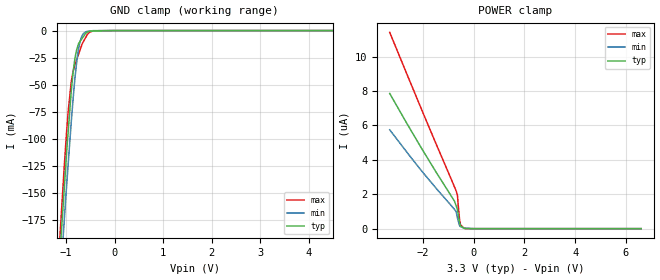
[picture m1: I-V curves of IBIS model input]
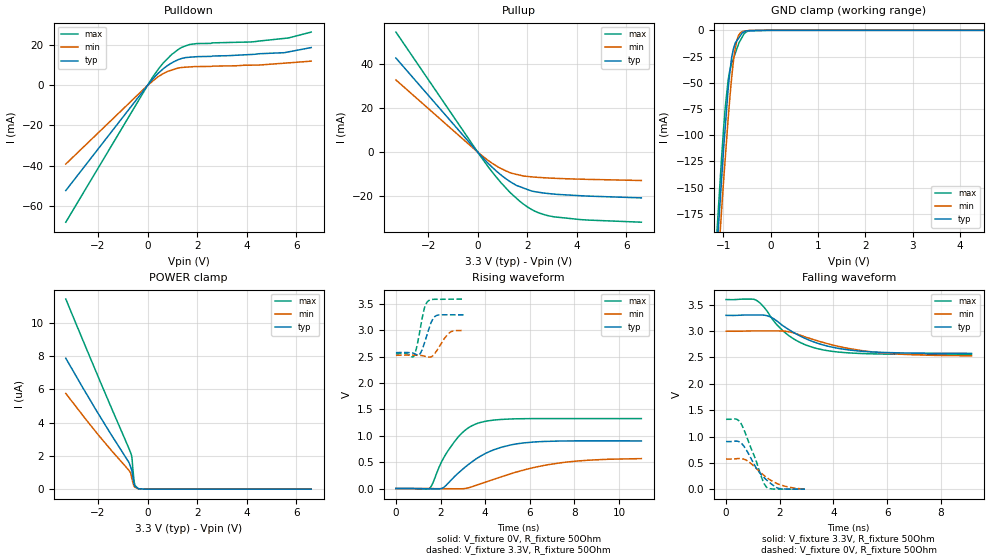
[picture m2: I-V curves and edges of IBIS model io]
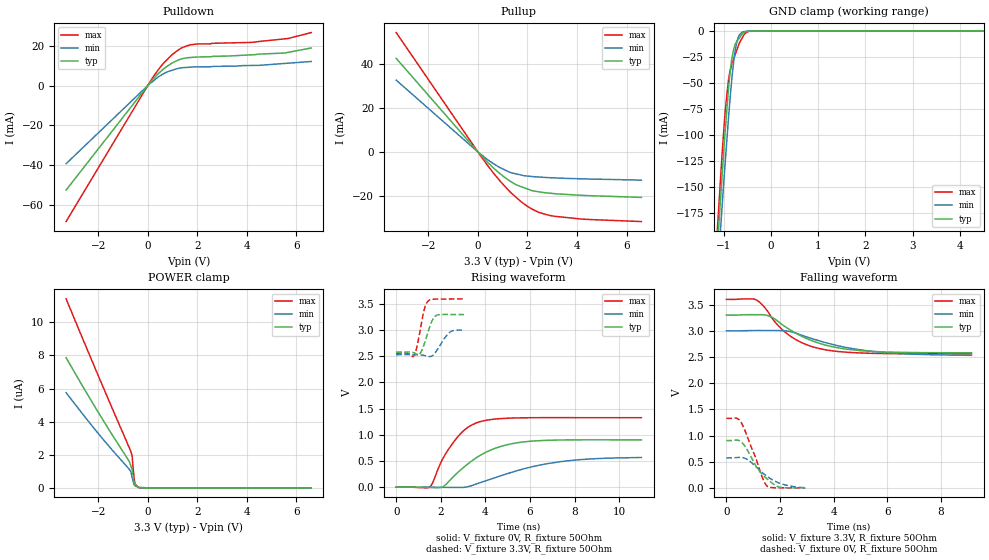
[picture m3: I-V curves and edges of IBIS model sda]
|Texas Instruments Incorporated
| 4ch/4ch Audio CODEC with 2Vrms Driver
| Marketing part#   Digital Voltage Range   Package-type   #pins
| PCM5310PAP   3.0V - 3.6V   HTQFP   64
| PCM5310PAPR   3.0V - 3.6V   HTQFP   64
[IBIS Ver]   3.2
[File name]   pcm5310.ibs
|SIMDE Ver   V3.0 - 201101 - RHL4 - Build 457
[File Rev]   1.0
[Date]   9/16/2011
[Source]
| Texas Instruments Incorporated.
| Analog-eLab Design Center, HPA
| 12500 TI Blvd
| Dallas, TX -75243
| e-mail: elab_scm_ibis@list.ti.com
[Notes]   Revision History:
| Rev 1.0: 9/16/2011
| - Initial version of the model
| - Model generated from simulations in TISPICE
| - Model matched to SPICE simulation
| - C_comp although listed in numerical order of value are
|   obtained from varying PVT conditions. For PVT conditions for
|   each specific value refer the buffer description under
|   respective [Model]. IBIS model user is responsible for using
|   appropriate C_comp to simulate for Signal Integrity.
[Disclaimer]
| This model is designed as an aid for customers of Texas Instruments.
| TI and its licensors and suppliers make no warranties, either expressed
| or implied, with respect to this  model, including the warranties of
| merchantability or fitness for a particular purpose. The model is
| provided solely on an "as is" basis. The entire risk as to its quality
| and performance is with the customer.
[Copyright]
 (C) Copyright 2011 Texas Instruments Incorporated.All rights reserved.
|   PCM5310
[Component]   PCM5310
[Manufacturer]   TI
[Package]   |64 HTQFP   -  PAP package
|   typ   min   max
R_pkg   0.15059   0.08833   0.17303
L_pkg   4.16735nH   3.79786nH   4.68209nH
C_pkg   0.68531pF   0.64149pF   0.80027pF
[Pin]  signal_name   model_name   R_pin   L_pin   C_pin
1   AIN1L   term   0.17241   4.66114nH  0.68445pF
2   AIN1R   term   0.16334   4.44486nH  0.72657pF
3   AIN2L   term   0.15617   4.26409nH  0.70301pF
4   AIN2R   term   0.15114   4.13963nH  0.68633pF
5   AIN3L   term   0.14796   4.05071nH  0.67300pF
6   AIN3R   term   0.14634   3.98580nH  0.66340pF
7   AIN4L   term   0.14631   3.95904nH  0.65785pF
8   AIN4R   term   0.14774   3.96845nH  0.65206pF
9   AIN5L   term   0.15083   4.02619nH  0.65642pF
10   AIN5R   term   0.15490   4.10975nH  0.66911pF
11   AIN6L   term   0.16036   4.24032nH  0.68311pF
12   AIN6R   term   0.16705   4.38885nH  0.68739pF
13   LO1L   term   0.15416   4.20529nH  0.68478pF
14   LO1R   term   0.15888   4.32238nH  0.70717pF
15   LO2L   term   0.16513   4.46842nH  0.72415pF
16   LO2R   term   0.17298   4.68209nH  0.68428pF
17   HGND   gnd   0.06388   3.97515nH  0.79207pF
18   VCCH   power   0.08669   3.91486nH  0.80765pF
19   HPOL   term   0.15364   4.22709nH  0.71008pF
20   VCCP   power   0.07930   3.59861nH  0.75747pF
21   PGND   gnd   0.05537   3.44453nH  0.77490pF
22   HPOR   term   0.14113   3.90151nH  0.66695pF
23   VCCDA   power   0.05352   3.30534nH  0.75554pF
24   AGNDDA   gnd   0.05323   3.27800nH  0.74902pF
25   VCOMDA   term   0.13754   3.79791nH  0.65288pF
26   AGNDS   gnd   0.07445   3.35983nH  0.70413pF
27   SDA   sda   0.13853   3.86286nH  0.65552pF
28   SCL   input   0.14155   3.94706nH  0.66652pF
29   SCK1   io   0.14535   4.05811nH  0.68452pF
30   BCK1   io   0.15232   4.21482nH  0.70298pF
31   LRCK1   io   0.15959   4.37814nH  0.72133pF
32   DATA1   io   0.17116   4.65573nH  0.68694pF
33   SCK2   io   0.17301   4.67994nH  0.68581pF
34   BCK2   io   0.16288   4.44274nH  0.72684pF
35   LRCK2   io   0.15655   4.27586nH  0.70407pF
36   DATA2   io   0.15089   4.13933nH  0.68651pF
37   SCK3   io   0.14816   4.05722nH  0.67339pF
38   BCK3   io   0.14632   3.98772nH  0.66321pF
39   LRCK3   io   0.14628   3.95934nH  0.65736pF
40   DATA3   io   0.14793   3.97169nH  0.64809pF
41   VDD   power   0.05593   3.39080nH  0.72906pF
42   DGND   gnd   0.05586   3.39760nH  0.74125pF
43   SCK4   io   0.14636   3.99488nH  0.66418pF
44   BCK4   io   0.14816   4.05714nH  0.67293pF
45   LRCK4   io   0.15096   4.15065nH  0.68929pF
46   DATA4   io   0.15661   4.28320nH  0.70608pF
47   SCK5   io   0.16282   4.42770nH  0.72281pF
48   BCK5   io   0.17303   4.68090nH  0.68810pF
49   LRCK5   io   0.17111   4.63717nH  0.68447pF
50   DATA5   io   0.15963   4.37847nH  0.72425pF
51   SCK6   io   0.15226   4.19368nH  0.69988pF
52   BCK6   io   0.14528   4.03450nH  0.68056pF
53   LRCK6   io   0.14153   3.93522nH  0.66613pF
54   DATA6   io   0.13849   3.84502nH  0.65470pF
55   GPIO1   io   0.13758   3.80184nH  0.64811pF
56   GPIO2   io   0.13828   3.79786nH  0.64149pF
57   GPIO3   io   0.14026   3.83554nH  0.64456pF
58   _RSTB   input   0.14434   3.91967nH  0.65643pF
59   AMUTE   input   0.14861   4.02993nH  0.66598pF
60   VCCAD   power   0.05705   3.53301nH  0.77678pF
61   AGNDAD   gnd   0.05818   3.62276nH  0.80355pF
62   VREFAD1   term   0.15708   4.28922nH  0.71633pF
63   VREFAD2   term   0.08833   3.95368nH  0.80027pF
64   VCOMAD   term   0.09223   4.14926nH  0.75899pF
[Model] term
Model_type Terminator
C_comp   1.0e-20F  1.0e-20F  1.0e-20F
|   typ   min   max
[Voltage Range]   3.3V   3.0V   3.6V
[POWER Clamp Reference]   3.3V   3.0V   3.6V
[GND Clamp Reference]   0V   0V   0V
|Ambient Temperature   25   85   -25
|Junction Temperature
[Temperature Range]   33   93   -25
| Models and submodels in the file (4): input (Input), io (I/O), sda (I/O), term (Terminator)
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|   input Model
[Model]   input
Model_type   Input
Vinl = 0.99
Vinh = 2.31
|   typ   min   max
|   (nom PVT)   (fast PVT)   (slow PVT)
C_comp   1.334e-12   1.158e-12   1.561e-12
| Where nom  PVT is Nominal Process, 3.3V, 33C
|   Fast PVT is Strong Process,  3.6V, -25C
|   Slow PVT is Weak Process,   3V, 93C
[Model Spec]
|Subparameter   typ   min   max
Vinh   2.31   2.1   2.52
Vinl   0.99   0.9   1.08
[Voltage Range]   3.3   3   3.6
|Ambient Temperature   25   85   -25
|Junction Temperature
[Temperature Range]   33   93   -25
[Power Clamp Reference]   3.3   3   3.6
[GND Clamp Reference]   0   0   0
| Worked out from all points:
|   GND clamp passes 1 mA (typ) near -0.54 V on its own axis
[GND Clamp]
|   Voltage   I(typ)   I(min)   I(max)
-3.3V     -1.899A    -1.874A    -1.956A
-1.149V   -221.5mA   -249.2mA   -204.1mA
-1.115V   -197mA     -226.3mA   -179.6mA
-1.048V   -150.6mA   -179.9mA   -130.2mA
-961.2mV  -94.27mA   -124.2mA   -75.24mA
-896.4mV  -56.08mA   -84.28mA   -47.17mA
-825mV    -26.82mA   -46.29mA   -31.99mA
-747mV    -12.19mA   -16.97mA   -21.98mA
-681mV    -7.826mA   -5.372mA   -13.54mA
-591mV    -2.011mA   -1.028mA   -5.715mA
-133.2mV  -132.3uA   -1.179uA   -14nA
6.6V      0A         0A         0A
[POWER Clamp]
|   Voltage   I(typ)   I(min)   I(max)
-3.3V     7.861uA    5.747uA    11.41uA
-2.046V   4.67uA     3.363uA    6.933uA
-745.8mV  1.586uA    1.113uA    2.411uA
-702mV    1.4uA      1.02uA     2.256uA
-678mV    1.298uA    947.2nA    2.16uA
-633.6mV  1.11uA     627.7nA    1.923uA
-601.2mV  803nA      442.6nA    1.326uA
-558mV    399.5nA    213.3nA    657nA
-518.4mV  190.8nA    121.1nA    267.6nA
-399.6mV  56.97nA    45.99nA    48.59nA
-133.2mV  0A         12.42nA    0A
6.6V      0A         0A         0A
|   io Model
[Model]   io
Model_type   I/O
Polarity   Non-Inverting
Enable   Active-Low
Vinl = 0.99
Vinh = 2.31
Vmeas = 1.65
Vref = 1.65
Cref = 20pF
Rref = 50
|   typ   min   max
|   (nom PVT)   (fast PVT)   (slow PVT)
C_comp   1.341e-12   1.164e-12   1.575e-12
|C_comp ON   1.391e-12   1.198e-12   1.650e-12
|C_comp High Z   1.292e-12   1.129e-12   1.501e-12
| Where nom  PVT is Nominal Process, 3.3V, 33C
|   Fast PVT is Strong Process,  3.6V, -25C
|   Slow PVT is Weak Process,   3V, 93C
[Model Spec]
|Subparameter   typ   min   max
Vinh   2.31   2.1   2.52
Vinl   0.99   0.9   1.08
[Voltage Range]   3.3   3   3.6
|Ambient Temperature   25   85   -25
|Junction Temperature
[Temperature Range]   33   93   -25
[Pullup Reference]   3.3   3   3.6
[Pulldown Reference]   0   0   0
[Power Clamp Reference]   3.3   3   3.6
[GND Clamp Reference]   0   0   0
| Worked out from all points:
|   slope of the pulldown table from 0 to 0.495 V, typ, clamps not added: 73.3 ohm
|   slope of the pullup table from 0 to 0.495 V, typ, clamps not added: 84.4 ohm
|   GND clamp passes 1 mA (typ) near -0.54 V on its own axis
|   falling waveform, V_fixture 3.3V, R_fixture 50Ohm: 20-80 % time 1.74ns typ, 2.29ns min, 1.33ns max; typ from 3.3 V to 2.58 V
|   rising waveform, V_fixture 0V, R_fixture 50Ohm: 20-80 % time 1.79ns typ, 2.89ns min, 1.18ns max; typ from 0 V to 0.904 V
|   rising waveform, V_fixture 3.3V, R_fixture 50Ohm: 20-80 % time 332ps typ, 442ps min, 284ps max; typ from 2.58 V to 3.29 V
|   falling waveform, V_fixture 0V, R_fixture 50Ohm: 20-80 % time 715ps typ, 863ps min, 575ps max; typ from 0.905 V to 0.001 V
[Pulldown]
|   Voltage   I(typ)   I(min)   I(max)
-3.3V     -52.46mA   -39.23mA   -68.24mA
172.8mV   2.65mA     1.778mA    3.487mA
586.8mV   7.767mA    5.542mA    10.48mA
979.2mV   11.22mA    7.635mA    15.45mA
1.382V    13.42mA    8.913mA    19mA
1.706V    14.03mA    9.196mA    20.41mA
2.578V    14.44mA    9.49mA     21.15mA
4.316V    15.47mA    10.08mA    21.78mA
5.674V    16.66mA    11.2mA     23.61mA
6.6V      18.83mA    12.06mA    26.55mA
[GND Clamp]
|   Voltage   I(typ)   I(min)   I(max)
-3.3V     -1.899A    -1.874A    -1.956A
-1.149V   -221.5mA   -249.2mA   -204.1mA
-1.115V   -197mA     -226.3mA   -179.6mA
-1.048V   -150.6mA   -179.9mA   -130.2mA
-961.2mV  -94.27mA   -124.2mA   -75.24mA
-896.4mV  -56.08mA   -84.28mA   -47.17mA
-825mV    -26.82mA   -46.29mA   -31.99mA
-747mV    -12.19mA   -16.97mA   -21.98mA
-681mV    -7.826mA   -5.372mA   -13.54mA
-591mV    -2.011mA   -1.028mA   -5.715mA
-133.2mV  -132.3uA   -1.179uA   -14nA
6.6V      0A         0A         0A
[Pullup]
|   Voltage   I(typ)   I(min)   I(max)
-3.3V     42.63mA    32.71mA    54.38mA
2.629fV   -176.6pA   -125.3pA   -192.6pA
396mV     -4.786mA   -3.572mA   -6.235mA
882mV     -9.807mA   -7.105mA   -13.09mA
1.246V    -12.9mA    -9.046mA   -17.57mA
1.574V    -15.12mA   -10.09mA   -21mA
1.825V    -16.16mA   -10.75mA   -23.37mA
2.168V    -17.59mA   -11.18mA   -25.92mA
2.473V    -18.19mA   -11.44mA   -27.55mA
3.089V    -19.01mA   -11.83mA   -29.31mA
4.316V    -19.84mA   -12.29mA   -30.67mA
6.6V      -20.71mA   -12.84mA   -31.72mA
[POWER Clamp]
|   Voltage   I(typ)   I(min)   I(max)
-3.3V     7.861uA    5.747uA    11.41uA
-2.046V   4.67uA     3.363uA    6.933uA
-745.8mV  1.586uA    1.113uA    2.411uA
-702mV    1.4uA      1.02uA     2.256uA
-678mV    1.298uA    947.2nA    2.16uA
-633.6mV  1.11uA     627.7nA    1.923uA
-601.2mV  803nA      442.6nA    1.326uA
-558mV    399.5nA    213.3nA    657nA
-518.4mV  190.8nA    121.1nA    267.6nA
-399.6mV  56.97nA    45.99nA    48.59nA
-133.2mV  0A         12.42nA    0A
6.6V      0A         0A         0A
[Ramp]
R_load = 50
|   typ   min   max
dV/dt_r   0.542102/1.79695e-09   0.340537/2.89024e-09   0.796156/1.17807e-09
dV/dt_f   0.432533/1.73934e-09   0.282327/2.30553e-09   0.625868/1.32736e-09
[Falling Waveform]
V_fixture = 3.3V
V_fixture_min = 3V
V_fixture_max = 3.6V
R_fixture = 50Ohm
|   Time   V(typ)   V(min)   V(max)
0s        3.3V       3V         3.6V
1.117ns   3.307V     3.006V     3.589V
1.427ns   3.303V     3.005V     3.446V
1.654ns   3.268V     3.005V     3.281V
2.344ns   3.028V     2.988V     2.913V
2.932ns   2.865V     2.893V     2.745V
3.533ns   2.75V      2.798V     2.653V
4.436ns   2.653V     2.684V     2.592V
5.837ns   2.596V     2.587V     2.565V
9.137ns   2.579V     2.531V     2.558V
[Rising Waveform]
V_fixture = 0V
V_fixture_min = 0V
V_fixture_max = 0V
R_fixture = 50Ohm
|   Time   V(typ)   V(min)   V(max)
0s        58.18uV    37.78uV    65.21uV
1.503ns   -5.332mV   49.14uV    3.119mV
2.112ns   14.01mV    -2.985mV   560.3mV
2.648ns   236mV      -4.539mV   902.6mV
3.169ns   428.9mV    5.399mV    1.129V
3.75ns    604.1mV    84mV       1.25V
4.724ns   782.5mV    222.4mV    1.311V
5.755ns   867.1mV    354.4mV    1.325V
7.72ns    903.1mV    505.4mV    1.328V
11ns      903.6mV    567.6mV    1.327V
[Rising Waveform]
V_fixture = 3.3V
V_fixture_min = 3V
V_fixture_max = 3.6V
R_fixture = 50Ohm
|   Time   V(typ)   V(min)   V(max)
0s        2.579V     2.529V     2.556V
800ps     2.566V     2.53V      2.51V
927ps     2.538V     2.529V     2.677V
1.104ns   2.571V     2.526V     3.064V
1.279ns   2.761V     2.513V     3.426V
1.438ns   2.978V     2.494V     3.556V
1.658ns   3.217V     2.522V     3.589V
1.833ns   3.285V     2.618V     3.591V
2.396ns   3.297V     2.956V     3.593V
3.041ns   3.295V     2.999V     3.595V
[Falling Waveform]
V_fixture = 0V
V_fixture_min = 0V
V_fixture_max = 0V
R_fixture = 50Ohm
|   Time   V(typ)   V(min)   V(max)
0s        904.6mV    572.8mV    1.327V
375ps     913.2mV    578.3mV    1.33V
552ps     879.9mV    581.6mV    1.25V
814ps     694.2mV    532.1mV    933mV
1.097ns   424.4mV    407.9mV    571.9mV
1.193ns   349.6mV    361.2mV    421.4mV
1.383ns   235.7mV    274.5mV    145.7mV
1.51ns    174.6mV    223.3mV    37.75mV
1.951ns   16.82mV    96.63mV    1.803mV
2.938ns   871.3uV    4.641mV    831.5uV
|   sda Model
[Model]   sda
Model_type   I/O
Polarity   Non-Inverting
Enable   Active-Low
Vinl = 0.99
Vinh = 2.31
Vmeas = 1.65
Vref = 1.65
Cref = 400pF
Rref = 50
|   typ   min   max
|   (nom PVT)   (fast PVT)   (slow PVT)
C_comp   1.341e-12   1.164e-12   1.575e-12
|C_comp ON   1.391e-12   1.198e-12   1.650e-12
|C_comp OFF   1.292e-12   1.129e-12   1.501e-12
| Where nom  PVT is Nominal Process, 3.3V, 33C
|   Fast PVT is Strong Process,  3.6V, -25C
|   Slow PVT is Weak Process,   3V, 93C
[Model Spec]
|Subparameter   typ   min   max
Vinh   2.31   2.1   2.52
Vinl   0.99   0.9   1.08
[Voltage Range]   3.3   3   3.6
|Ambient Temperature   25   85   -25
|Junction Temperature
[Temperature Range]   33   93   -25
[Pullup Reference]   3.3   3   3.6
[Pulldown Reference]   0   0   0
[Power Clamp Reference]   3.3   3   3.6
[GND Clamp Reference]   0   0   0
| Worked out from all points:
|   slope of the pulldown table from 0 to 0.495 V, typ, clamps not added: 73.3 ohm
|   slope of the pullup table from 0 to 0.495 V, typ, clamps not added: 84.4 ohm
|   GND clamp passes 1 mA (typ) near -0.54 V on its own axis
|   falling waveform, V_fixture 3.3V, R_fixture 50Ohm: 20-80 % time 1.74ns typ, 2.29ns min, 1.33ns max; typ from 3.3 V to 2.58 V
|   rising waveform, V_fixture 0V, R_fixture 50Ohm: 20-80 % time 1.79ns typ, 2.89ns min, 1.18ns max; typ from 0 V to 0.904 V
|   rising waveform, V_fixture 3.3V, R_fixture 50Ohm: 20-80 % time 332ps typ, 442ps min, 284ps max; typ from 2.58 V to 3.29 V
|   falling waveform, V_fixture 0V, R_fixture 50Ohm: 20-80 % time 715ps typ, 863ps min, 575ps max; typ from 0.905 V to 0.001 V
[Pulldown]
|   Voltage   I(typ)   I(min)   I(max)
-3.3V     -52.46mA   -39.23mA   -68.24mA
172.8mV   2.65mA     1.778mA    3.487mA
586.8mV   7.767mA    5.542mA    10.48mA
979.2mV   11.22mA    7.635mA    15.45mA
1.382V    13.42mA    8.913mA    19mA
1.706V    14.03mA    9.196mA    20.41mA
2.578V    14.44mA    9.49mA     21.15mA
4.316V    15.47mA    10.08mA    21.78mA
5.674V    16.66mA    11.2mA     23.61mA
6.6V      18.83mA    12.06mA    26.55mA
[GND Clamp]
|   Voltage   I(typ)   I(min)   I(max)
-3.3V     -1.899A    -1.874A    -1.956A
-1.149V   -221.5mA   -249.2mA   -204.1mA
-1.115V   -197mA     -226.3mA   -179.6mA
-1.048V   -150.6mA   -179.9mA   -130.2mA
-961.2mV  -94.27mA   -124.2mA   -75.24mA
-896.4mV  -56.08mA   -84.28mA   -47.17mA
-825mV    -26.82mA   -46.29mA   -31.99mA
-747mV    -12.19mA   -16.97mA   -21.98mA
-681mV    -7.826mA   -5.372mA   -13.54mA
-591mV    -2.011mA   -1.028mA   -5.715mA
-133.2mV  -132.3uA   -1.179uA   -14nA
6.6V      0A         0A         0A
[Pullup]
|   Voltage   I(typ)   I(min)   I(max)
-3.3V     42.63mA    32.71mA    54.38mA
2.629fV   -176.6pA   -125.3pA   -192.6pA
396mV     -4.786mA   -3.572mA   -6.235mA
882mV     -9.807mA   -7.105mA   -13.09mA
1.246V    -12.9mA    -9.046mA   -17.57mA
1.574V    -15.12mA   -10.09mA   -21mA
1.825V    -16.16mA   -10.75mA   -23.37mA
2.168V    -17.59mA   -11.18mA   -25.92mA
2.473V    -18.19mA   -11.44mA   -27.55mA
3.089V    -19.01mA   -11.83mA   -29.31mA
4.316V    -19.84mA   -12.29mA   -30.67mA
6.6V      -20.71mA   -12.84mA   -31.72mA
[POWER Clamp]
|   Voltage   I(typ)   I(min)   I(max)
-3.3V     7.861uA    5.747uA    11.41uA
-2.046V   4.67uA     3.363uA    6.933uA
-745.8mV  1.586uA    1.113uA    2.411uA
-702mV    1.4uA      1.02uA     2.256uA
-678mV    1.298uA    947.2nA    2.16uA
-633.6mV  1.11uA     627.7nA    1.923uA
-601.2mV  803nA      442.6nA    1.326uA
-558mV    399.5nA    213.3nA    657nA
-518.4mV  190.8nA    121.1nA    267.6nA
-399.6mV  56.97nA    45.99nA    48.59nA
-133.2mV  0A         12.42nA    0A
6.6V      0A         0A         0A
[Ramp]
R_load = 50
|   typ   min   max
dV/dt_r   0.542102/1.79695e-09   0.340537/2.89024e-09   0.796156/1.17807e-09
dV/dt_f   0.432533/1.73934e-09   0.282327/2.30553e-09   0.625868/1.32736e-09
[Falling Waveform]
V_fixture = 3.3V
V_fixture_min = 3V
V_fixture_max = 3.6V
R_fixture = 50Ohm
|   Time   V(typ)   V(min)   V(max)
0s        3.3V       3V         3.6V
1.117ns   3.307V     3.006V     3.589V
1.427ns   3.303V     3.005V     3.446V
1.654ns   3.268V     3.005V     3.281V
2.344ns   3.028V     2.988V     2.913V
2.932ns   2.865V     2.893V     2.745V
3.533ns   2.75V      2.798V     2.653V
4.436ns   2.653V     2.684V     2.592V
5.837ns   2.596V     2.587V     2.565V
9.137ns   2.579V     2.531V     2.558V
[Rising Waveform]
V_fixture = 0V
V_fixture_min = 0V
V_fixture_max = 0V
R_fixture = 50Ohm
|   Time   V(typ)   V(min)   V(max)
0s        58.18uV    37.78uV    65.21uV
1.503ns   -5.332mV   49.14uV    3.119mV
2.112ns   14.01mV    -2.985mV   560.3mV
2.648ns   236mV      -4.539mV   902.6mV
3.169ns   428.9mV    5.399mV    1.129V
3.75ns    604.1mV    84mV       1.25V
4.724ns   782.5mV    222.4mV    1.311V
5.755ns   867.1mV    354.4mV    1.325V
7.72ns    903.1mV    505.4mV    1.328V
11ns      903.6mV    567.6mV    1.327V
[Rising Waveform]
V_fixture = 3.3V
V_fixture_min = 3V
V_fixture_max = 3.6V
R_fixture = 50Ohm
|   Time   V(typ)   V(min)   V(max)
0s        2.579V     2.529V     2.556V
800ps     2.566V     2.53V      2.51V
927ps     2.538V     2.529V     2.677V
1.104ns   2.571V     2.526V     3.064V
1.279ns   2.761V     2.513V     3.426V
1.438ns   2.978V     2.494V     3.556V
1.658ns   3.217V     2.522V     3.589V
1.833ns   3.285V     2.618V     3.591V
2.396ns   3.297V     2.956V     3.593V
3.041ns   3.295V     2.999V     3.595V
[Falling Waveform]
V_fixture = 0V
V_fixture_min = 0V
V_fixture_max = 0V
R_fixture = 50Ohm
|   Time   V(typ)   V(min)   V(max)
0s        904.6mV    572.8mV    1.327V
375ps     913.2mV    578.3mV    1.33V
552ps     879.9mV    581.6mV    1.25V
814ps     694.2mV    532.1mV    933mV
1.097ns   424.4mV    407.9mV    571.9mV
1.193ns   349.6mV    361.2mV    421.4mV
1.383ns   235.7mV    274.5mV    145.7mV
1.51ns    174.6mV    223.3mV    37.75mV
1.951ns   16.82mV    96.63mV    1.803mV
2.938ns   871.3uV    4.641mV    831.5uV
